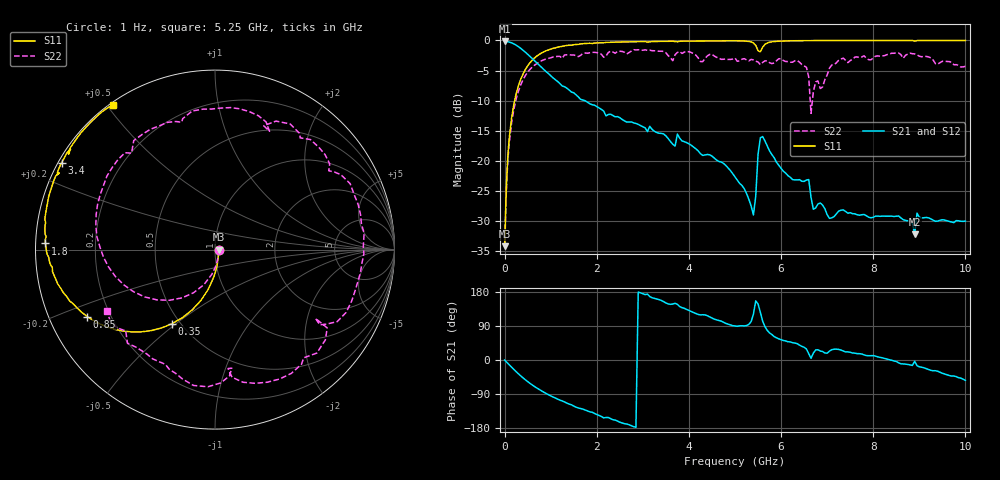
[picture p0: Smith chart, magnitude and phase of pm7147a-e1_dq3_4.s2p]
# GHz S DB R 50
! S-Parameters data
! Freq  dbS11  angS11  dbS21  angS21  dbS12  angS12  dbS22  angS22
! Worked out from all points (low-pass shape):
!   279 points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, 1 Hz to 10 GHz, reference 50 ohm
!   highest |S21| = -0.17 dB at 7.9 Hz (marker M1); lowest = -32.2 dB at 8.9 GHz (marker M2)
!   |S21| within 3 dB of the highest: start of sweep to 621.4 MHz
!   lowest |S11| = -34.2 dB at 1.995 kHz (marker M3), VSWR 1.04, Z = 52 - j0.00031 ohm
!   |S11| at or under -10 dB: start of sweep to 218.2 MHz
!   |S22| runs from -34.2 to -1.5 dB; largest |S21 - S12| = 0
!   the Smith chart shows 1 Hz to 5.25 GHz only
!   S11 on the Smith chart (normalised r, x): 1 Hz: 1.04, -0.00; 350 MHz: 0.45, -0.48; 850 MHz: 0.12, -0.24; 1.8 GHz: 0.03, +0.02; 3.4 GHz: 0.01, +0.26; 5.25 GHz: 0.01, +0.52
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1e-09  -34.17 -0.0  -0.17 -0.0  -0.17 -0.0  -34.17 -0.0
7.9e-09  -34.17 -0.0  -0.17 -0.0  -0.17 -0.0  -34.17 -0.0
1.9953e-06  -34.17 -0.0  -0.17 -0.0  -0.17 -0.0  -34.17 -0.0
0.1  -16.33 -92.5  -0.28 -12.6  -0.28 -12.6  -17.11 -97.4
0.35  -6.45 -120.0  -1.32 -41.9  -1.32 -41.9  -7.37 -139.1
0.85  -1.90 -152.3  -4.82 -84.9  -4.82 -84.9  -3.22 163.6
1.7  -0.54 -179.7  -9.90 -129.6  -9.90 -129.6  -2.13 99.3
1.8  -0.49 177.9  -10.26 -134.5  -10.26 -134.5  -2.12 91.4
2.75  -0.23 160.2  -13.53 -173.2  -13.53 -173.2  -1.76 30.7
3.35  -0.16 151.2  -15.41 159.4  -15.41 159.4  -1.79 -16.7
3.4  -0.16 150.5  -15.44 157.3  -15.44 157.3  -1.79 -20.6
4.1  -0.10 141.3  -17.69 125.2  -17.69 125.2  -2.18 -73.3
5.05  -0.07 128.8  -23.24 89.0  -23.24 89.0  -3.46 -137.9
5.25  -0.12 125.3  -25.41 90.8  -25.41 90.8  -3.23 -150.5
5.4  -0.42 121.1  -28.98 121.0  -28.98 121.0  -3.23 -160.1
5.6  -1.14 130.5  -15.96 102.4  -15.96 102.4  -3.66 -167.9
6.55  -0.05 116.5  -23.18 29.1  -23.18 29.1  -4.47 124.5
6.7  -0.03 115.1  -28.03 18.2  -28.03 18.2  -8.54 150.3
7.25  -0.01 110.0  -28.34 28.0  -28.34 28.0  -3.30 132.9
8.35  -0.01 101.0  -29.18 1.1  -29.18 1.1  -2.24 78.9
8.9  -0.12 96.1  -32.21 -3.3  -32.21 -3.3  -2.24 48.2
10  -0.01 89.9  -30.01 -53.8  -30.01 -53.8  -4.31 -19.4
